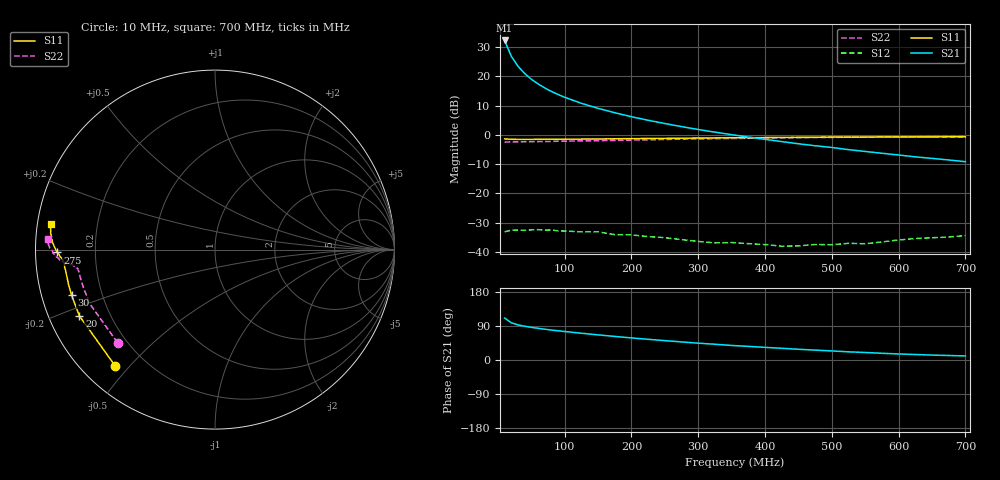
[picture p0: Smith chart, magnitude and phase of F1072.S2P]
! Date: Mon Aug 07 16:36:22 1995
# MHZ  S  MA  R  50.0000
!  POLYFET RF DEVICES
!  F1072 (Each Side)
!  S PARAMETERS
!  VDS=28V, IDQ=600mA
!FREQ  S11MAG S11ANG S21MAG S21ANG S12MAG S12ANG S22MAG S22ANG
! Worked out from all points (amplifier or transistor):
!   34 points, 10 MHz to 700 MHz, reference 50 ohm
!   highest |S21| = 32.3 dB at 10 MHz (marker M1)
!   |S21| within 3 dB of that: start of sweep to 15.54 MHz
!   unconditionally stable (mu >= 1): 296.4 MHz to end of sweep
!   at 60 MHz: K = 0.16, MSG = 24.9 dB, |S12| = -32.4 dB
!   at 300 MHz: K = 1.02, MAG = 18.2 dB, |S12| = -36.5 dB
!   at 700 MHz: K = 1.22, MAG = 9.8 dB, |S12| = -34.5 dB
!   S11 on the Smith chart (normalised r, x): 10 MHz: 0.10, -0.46; 20 MHz: 0.09, -0.23; 30 MHz: 0.09, -0.15; 275 MHz: 0.06, -0.01; 700 MHz: 0.04, +0.08
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10  0.8537 -130.7  41.31 110.9  0.02192 23.8  0.7508 -136.3
20  0.8409 -154.0  22.15 98.2  0.02342 9.6  0.7605 -156.7
30  0.8384 -162.5  14.93 92.7  0.02348 6.1  0.7629 -163.7
40  0.8389 -166.7  11.23 89.1  0.02332 2.5  0.7654 -167.1
50  0.8385 -169.3  8.979 86.1  0.02365 1.9  0.7674 -169.3
60  0.8402 -171.1  7.463 83.6  0.02388 0.6  0.7685 -170.7
70  0.8407 -172.3  6.374 81.2  0.02347 -0.4  0.7706 -171.5
80  0.8439 -173.2  5.549 79.1  0.02359 -1.1  0.7725 -172.3
90  0.843 -173.8  4.916 77.1  0.02279 -2.1  0.7787 -172.5
100  0.8434 -174.5  4.404 75.2  0.02261 -3.3  0.7792 -172.8
125  0.8477 -175.5  3.471 70.6  0.02189 -4.6  0.7919 -173.4
150  0.8498 -176.3  2.846 66.3  0.02196 -5.2  0.7965 -173.8
175  0.8577 -177.0  2.395 62.2  0.01964 -5.9  0.8047 -174.1
200  0.8631 -177.3  2.045 58.3  0.01945 -7.6  0.8148 -174.1
250  0.8722 -178.5  1.563 51.1  0.01741 -5.8  0.8347 -174.9
275  0.8784 -179.0  1.387 47.7  0.01613 -4.9  0.8457 -175.2
325  0.8871 180.0  1.114 41.6  0.01418 -1.4  0.8635 -176.0
375  0.8973 178.8  0.9161 35.9  0.01378 9.9  0.8741 -176.9
425  0.9053 177.7  0.768 30.9  0.01246 18.1  0.8923 -178.0
475  0.9095 176.5  0.6518 26.1  0.01332 27.6  0.9041 -178.9
600  0.9203 173.7  0.4526 16.0  0.01591 48.9  0.9257 178.6
700  0.9277 171.0  0.3478 10.8  0.01893 57.1  0.9339 176.2
